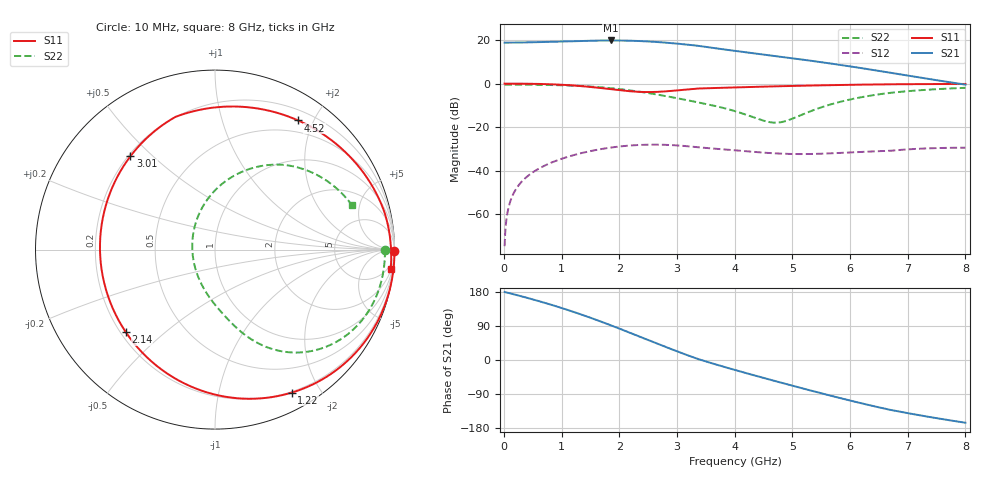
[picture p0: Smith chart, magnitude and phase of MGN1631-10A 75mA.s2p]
! Port[1] = GATE
! Port[2] = DRAIN
! [Type]  S-parameter s2p file touchstone ver. 1.0
! [Object]  MGN1631-10A
! [Bias]  75 mA
! [Version]  1.0
! [Date]  Thu May 19 10:12:30 2026
! [Source]  This file was created in JSC "ICC Milandr".
! [Disclaimer] Property of JSC "ICC Milandr". Unauthorized reproduction and/or distribution is strictly prohibited.
!  The file and the data are provided "AS IS" and with all faults and disclaim all warranties, express and implied, including
!  without limitation any implied warranties of merchantability, fitness for a particular purpose.
!  JSC "ICC Milandr" assumes no liability for:
!  1) the accuracy of the data provided;
!  2) the proper functioning of this data;
!  3) infringement of patents, copyrights or intellectual property rights resulting from the use of this data.
!  JSC "ICC Milandr" reserves the right to make changes to the products and the data without prior notice.
!  Please, be aware that your receipt and use of the file provided shall serve as acceptance of these terms and conditions.
!  If you do not accept these terms, you should return or destroy this file and any other accompanying information immediately.
# Hz S MA R 12.5
! freq  S11mag  S11ang  S21mag  S21ang  S12mag  S12ang  S22mag  S22ang
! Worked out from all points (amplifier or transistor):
!   800 points, 10 MHz to 8 GHz, reference 12.5 ohm
!   highest |S21| = 19.9 dB at 1.85 GHz (marker M1)
!   |S21| within 3 dB of that: start of sweep to 3.507 GHz
!   unconditionally stable (mu >= 1): 4.191 GHz to 5.382 GHz
!   at 1.34 GHz: K = 0.34, MSG = 25.8 dB, |S12| = -32.0 dB
!   at 4.01 GHz: K = 0.96, MSG = 22.9 dB, |S12| = -30.7 dB
!   at 8 GHz: K = 0.38, MSG = 14.5 dB, |S12| = -29.5 dB
!   S11 on the Smith chart (normalised r, x): 10 MHz: open; 1.22 GHz: 0.19, -1.65; 2.14 GHz: 0.22, -0.37; 3.01 GHz: 0.21, +0.43; 4.52 GHz: 0.33, +1.78; 8 GHz: 2, -18
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1e7  1 -0.4  8.806 179.5  0.0001818 85.4  0.9468 -0.2
8e7  1 -3.6  8.794 176.9  0.001443 86.9  0.9472 -1.7
1.9e8  1 -8.5  8.816 172.6  0.003433 83.7  0.9471 -4.2
6.8e8  0.9798 -31.6  9.091 152.0  0.01252 66.9  0.9371 -15.3
9.6e8  0.9486 -46.5  9.327 139.1  0.0179 56.1  0.921 -22.0
1.22e9  0.904 -61.9  9.553 126.2  0.02291 45.3  0.8963 -28.6
1.35e9  0.876 -70.3  9.655 119.5  0.02537 39.6  0.8797 -32.1
1.61e9  0.8108 -89.1  9.812 105.3  0.03002 27.6  0.8373 -39.1
1.85e9  0.7457 -109.2  9.865 91.7  0.03379 16.0  0.7868 -45.6
2.14e9  0.677 -137.3  9.766 74.5  0.03726 1.3  0.7126 -53.5
2.39e9  0.6441 -164.2  9.516 59.4  0.03901 -11.6  0.6406 -60.0
2.68e9  0.6494 164.2  9.04 41.8  0.0394 -26.4  0.5539 -66.8
3.01e9  0.7016 132.2  8.319 22.4  0.03781 -42.7  0.4599 -74.0
3.25e9  0.7526 112.9  7.731 8.8  0.03555 -53.9  0.398 -79.2
3.47e9  0.7799 99.0  7.094 -2.4  0.0334 -61.6  0.3477 -84.5
4.01e9  0.8193 74.2  5.665 -26.6  0.02902 -71.2  0.232 -104.4
4.52e9  0.8557 57.2  4.633 -48.1  0.0257 -72.5  0.1382 -148.3
4.91e9  0.8811 46.8  3.976 -64.1  0.02422 -69.1  0.1412 151.6
5.34e9  0.9067 36.9  3.34 -81.5  0.02408 -63.0  0.2386 108.4
5.98e9  0.9395 24.2  2.522 -106.2  0.02609 -56.2  0.4263 75.4
6.67e9  0.9672 12.3  1.806 -130.7  0.02822 -55.2  0.6085 50.9
8e9  0.9849 -6.3  0.9495 -165.6  0.0336 -78.1  0.8017 18.1
